|   IBIS model for TI xxx DSP
[IBIS Ver]   5.1
[Disclaimer]   Please be aware that in the absence of a written agreement
|   Texas Instruments(TI) assumes no liability for:
|   (1) The accuracy of the IBIS models provided to your company,
|   however, the IBIS model is compliant to industry standard
|   IQ Level 2a.  Refer to IBIS Quality Section below for
|   for full details.
|   (2) The proper functioning of these Models in your design
|   or for any resulting applications
|   (3) Infringement of patents, copyrights or intellectual
|   property rights resulting from your use of these
|   models.
|   TI provides IBIS Models as a service to our customers and
|   therefore reserves the right to limit distribution of the
|   Models.  The information is subject to change without notice.
[File Name]  sprm785c.ibs
[File Rev]   0.4
|   - Initial version
|   - Fixed typo in I/O assignment
|   - Removed unsupported SDIO/LVCMOS drive strengths
|   - Updated with supported drive strengths for IIC and eMMC buffers
[Date]   26 Oct 2023
[Source]   Texas Instruments Incorporated
[Copyright]   Property of Texas Instruments Incorporated.
|   Unauthorized reproduction and/or distribution is strictly.
|   prohibited.
|   This product is protected under copyright law and trade
|   secret law as an unpublished work.
|   Created 2012,(C) Copyright 1999-2012,
|   Texas Instruments Incorporated., All Rights Reserved.
|   These commodities are under the U.S. Government
|   distribution license control. As such,they are not to be
|   re-exported without the prior approval of the U.S.
|   Department of Commerce.
[Notes]
   This file does not include AMI models for SerDes based links.
   For SerDes simulations use Texas Instruments IBIS AMI models
   Some IV curves contain Non monotonic data points.
|   Revision History
|   GERNERAL COMMENT: All IBIS Quality Notes below reflect latest release
|   and version of IBIS File
|   File passes ibischk5.1 and ibischk6 with 0 errors and 200 warnings
|   Component AM62A
[Component] AM62A
[Manufacturer] Texas Instruments
[Package]
|   typ   min   max
R_pkg   0.40877   0.11887   0.72369
L_pkg   2.422e-9   9.157e-10   3.836e-9
C_pkg   1.228e-12   5.686e-13   1.785e-12
[Package Model]   am62a_pkg
[Pin]	Signal_name	model_name
E7	ATEST0	NC
V11	CSI0_ATB_0_H	NC
U11	CSI0_ATB_1_H	NC
AB14	CSI0_RXCLKN	NC
AB13	CSI0_RXCLKP	NC
W12	CSI0_RXN0	NC
Y13	CSI0_RXN1	NC
AA13	CSI0_RXN2	NC
AB11	CSI0_RXN3	NC
W13	CSI0_RXP0	NC
Y14	CSI0_RXP1	NC
AA12	CSI0_RXP2	NC
AB10	CSI0_RXP3	NC
V10	CSI0_RXRCALIB	NC
J5	DDR0_A0		DDR_SE
J2	DDR0_A1		DDR_SE
K2	DDR0_A10	DDR_SE
L5	DDR0_A11	DDR_SE
M3	DDR0_A12	DDR_SE
M2	DDR0_A13	DDR_SE
J4	DDR0_A2		DDR_SE
L4	DDR0_A3		DDR_SE
J1	DDR0_A4		DDR_SE
K5	DDR0_A5		DDR_SE
K3	DDR0_A6		DDR_SE
H2	DDR0_A7		DDR_SE
L6	DDR0_A8		DDR_SE
L2	DDR0_A9		DDR_SE
N5	DDR0_ACT_N	DDR_SE
H7	DDR0_ALERT_N	DDR_SE
G7	DDR0_ATB0	DDR_SE
F6	DDR0_ATB1	DDR_SE
K6	DDR0_BA0	DDR_SE
H3	DDR0_BA1	DDR_SE
P4	DDR0_BG0	DDR_SE
R7	DDR0_BG1	DDR_SE
H6	DDR0_CAL0	DDR_SE
M5	DDR0_CAS_N	DDR_SE
M1	DDR0_CK0	DDR_DIFF_P
L1	DDR0_CK0_N	DDR_DIFF_N
P3	DDR0_CKE0	DDR_SE
P5	DDR0_CKE1	DDR_SE
J6	DDR0_CS0_N	DDR_SE
N4	DDR0_CS1_N	DDR_SE
C2	DDR0_DM0	DDR_SE
F3	DDR0_DM1	DDR_SE
U1	DDR0_DM2	DDR_SE
W3	DDR0_DM3	DDR_SE
A5	DDR0_DQ0	DDR_SE
B4	DDR0_DQ1	DDR_SE
E6	DDR0_DQ10	DDR_SE
G2	DDR0_DQ11	DDR_SE
G6	DDR0_DQ12	DDR_SE
G4	DDR0_DQ13	DDR_SE
E4	DDR0_DQ14	DDR_SE
D3	DDR0_DQ15	DDR_SE
T6	DDR0_DQ16	DDR_SE
T4	DDR0_DQ17	DDR_SE
U5	DDR0_DQ18	DDR_SE
R5	DDR0_DQ19	DDR_SE
B6	DDR0_DQ2	DDR_SE
P2	DDR0_DQ20	DDR_SE
R3	DDR0_DQ21	DDR_SE
T2	DDR0_DQ22	DDR_SE
U3	DDR0_DQ23	DDR_SE
Y2	DDR0_DQ24	DDR_SE
V2	DDR0_DQ25	DDR_SE
V4	DDR0_DQ26	DDR_SE
W5	DDR0_DQ27	DDR_SE
Y4	DDR0_DQ28	DDR_SE
AA3	DDR0_DQ29	DDR_SE
D5	DDR0_DQ3	DDR_SE
AA5	DDR0_DQ30	DDR_SE
AB4	DDR0_DQ31	DDR_SE
C5	DDR0_DQ4	DDR_SE
C3	DDR0_DQ5	DDR_SE
B2	DDR0_DQ6	DDR_SE
A3	DDR0_DQ7	DDR_SE
E2	DDR0_DQ8	DDR_SE
F5	DDR0_DQ9	DDR_SE
D1	DDR0_DQS0	DDR_DIFF_P
C1	DDR0_DQS0_N	DDR_DIFF_N
G1	DDR0_DQS1	DDR_DIFF_P
F1	DDR0_DQS1_N	DDR_DIFF_N
R1	DDR0_DQS2	DDR_DIFF_P
P1	DDR0_DQS2_N	DDR_DIFF_N
W1	DDR0_DQS3	DDR_DIFF_P
Y1	DDR0_DQS3_N	DDR_DIFF_N
H5	DDR0_ODT0	DDR_SE
N3	DDR0_ODT1	DDR_SE
N2	DDR0_PAR	DDR_SE
M6	DDR0_RAS_N	DDR_SE
P6	DDR0_RESET0_N	DDR_SE
N6	DDR0_WE_N	DDR_SE
C13	EMU0		LVCMOS_V
E10	EMU1		LVCMOS_V
B16	EXT_REFCLK1	LVCMOS_V
F17	EXTINTN		IIC_V
N21	GPMC0_AD0	LVCMOS_H
N20	GPMC0_AD1	LVCMOS_H
R20	GPMC0_AD10	LVCMOS_H
R22	GPMC0_AD11	LVCMOS_H
T22	GPMC0_AD12	LVCMOS_H
R21	GPMC0_AD13	LVCMOS_H
T20	GPMC0_AD14	LVCMOS_H
T21	GPMC0_AD15	LVCMOS_H
N19	GPMC0_AD2	LVCMOS_H
N18	GPMC0_AD3	LVCMOS_H
N17	GPMC0_AD4	LVCMOS_H
P18	GPMC0_AD5	LVCMOS_H
P19	GPMC0_AD6	LVCMOS_H
P21	GPMC0_AD7	LVCMOS_H
P22	GPMC0_AD8	LVCMOS_H
R19	GPMC0_AD9	LVCMOS_H
L18	GPMC0_ADVN_ALE	LVCMOS_H
L19	GPMC0_BE0N_CLE	LVCMOS_H
M18	GPMC0_BE1N	LVCMOS_H
N22	GPMC0_CLK	LVCMOS_H
M19	GPMC0_CSN0	LVCMOS_H
M21	GPMC0_CSN1	LVCMOS_H
M22	GPMC0_CSN2	LVCMOS_H
M20	GPMC0_CSN3	LVCMOS_H
K18	GPMC0_DIR	LVCMOS_H
L17	GPMC0_OEN_REN	LVCMOS_H
R18	GPMC0_WAIT0	LVCMOS_H
R17	GPMC0_WAIT1	LVCMOS_H
K19	GPMC0_WEN	LVCMOS_H
K17	GPMC0_WPN	LVCMOS_H
D17	I2C0_SCL	LVCMOS_V
E16	I2C0_SDA	LVCMOS_V
C17	I2C1_SCL	LVCMOS_V
E17	I2C1_SDA	LVCMOS_V
C6	IFORCE		NC
C18	MCAN0_RX	LVCMOS_V
B17	MCAN0_TX	LVCMOS_V
A21	MCASP0_ACLKR	LVCMOS_V
A19	MCASP0_ACLKX	LVCMOS_V
B21	MCASP0_AFSR	LVCMOS_V
A20	MCASP0_AFSX	LVCMOS_V
B20	MCASP0_AXR0	LVCMOS_V
B18	MCASP0_AXR1	LVCMOS_V
B19	MCASP0_AXR2	LVCMOS_V
C19	MCASP0_AXR3	LVCMOS_V
B8	MCU_ERRORN	LVCMOS_H
E12	MCU_I2C0_SCL	IIC_V
D9	MCU_I2C0_SDA	IIC_V
E8	MCU_MCAN0_RX	LVCMOS_V
C7	MCU_MCAN0_TX	LVCMOS_V
B9	MCU_MCAN1_RX	LVCMOS_V
D7	MCU_MCAN1_TX	LVCMOS_V
A12	MCU_OSC0_XI	NC
A11	MCU_OSC0_XO	NC
A7	MCU_PORZ	RESET_H
D14	MCU_RESETSTATZ	LVCMOS_V
C12	MCU_RESETZ	LVCMOS_V
B13	MCU_SPI0_CLK	LVCMOS_V
E11	MCU_SPI0_CS0	LVCMOS_V
C11	MCU_SPI0_CS1	LVCMOS_V
A15	MCU_SPI0_D0	LVCMOS_V
B12	MCU_SPI0_D1	LVCMOS_V
B11	MCU_UART0_CTSN	LVCMOS_V
D10	MCU_UART0_RTSN	LVCMOS_V
D8	MCU_UART0_RXD	LVCMOS_V
F8	MCU_UART0_TXD	LVCMOS_V
V12	MDIO0_MDC	LVCMOS_V
V13	MDIO0_MDIO	LVCMOS_V
AB7	MMC0_CLK	SDIO_V
Y6	MMC0_CMD	SDIO_V
AA6	MMC0_DAT0	SDIO_V
AB6	MMC0_DAT1	SDIO_V
Y7	MMC0_DAT2	SDIO_V
AA7	MMC0_DAT3	SDIO_V
Y8	MMC0_DAT4	SDIO_V
W7	MMC0_DAT5	SDIO_V
W9	MMC0_DAT6	SDIO_V
AB8	MMC0_DAT7	SDIO_V
E22	MMC1_CLK	SDIO_V
C21	MMC1_CMD	SDIO_V
B22	MMC1_DAT0	SDIO_V
D21	MMC1_DAT1	SDIO_V
C22	MMC1_DAT2	SDIO_V
D22	MMC1_DAT3	SDIO_V
E18	MMC1_SDCD	LVCMOS_V
D18	MMC1_SDWP	LVCMOS_V
H22	MMC2_CLK	SDIO_H
G22	MMC2_CMD	SDIO_H
E20	MMC2_DAT0	SDIO_H
F21	MMC2_DAT1	SDIO_H
F20	MMC2_DAT2	SDIO_H
G21	MMC2_DAT3	SDIO_H
F22	MMC2_SDCD	LVCMOS_H
E21	MMC2_SDWP	LVCMOS_H
L22	OSPI0_CLK	LVCMOS_H
H21	OSPI0_CSN0	LVCMOS_H
G19	OSPI0_CSN1	LVCMOS_H
K20	OSPI0_CSN2	LVCMOS_H
G20	OSPI0_CSN3	LVCMOS_H
J21	OSPI0_D0	LVCMOS_H
J18	OSPI0_D1	LVCMOS_H
J19	OSPI0_D2	LVCMOS_H
H18	OSPI0_D3	LVCMOS_H
K21	OSPI0_D4	LVCMOS_H
H19	OSPI0_D5	LVCMOS_H
J20	OSPI0_D6	LVCMOS_H
J22	OSPI0_D7	LVCMOS_H
L21	OSPI0_DQS	LVCMOS_H
K22	OSPI0_LBCLKO	LVCMOS_H
D12	PMIC_LPM_EN0	LVCMOS_V
F18	PORZ_OUT	LVCMOS_V
E19	RESET_REQZ	LVCMOS_V
F19	RESETSTATZ	LVCMOS_V
AB16	RGMII1_RD0	LVCMOS_V
V15	RGMII1_RD1	LVCMOS_V
W15	RGMII1_RD2	LVCMOS_V
V14	RGMII1_RD3	LVCMOS_V
AA15	RGMII1_RX_CTL	LVCMOS_V
AA16	RGMII1_RXC	LVCMOS_V
Y17	RGMII1_TD0	LVCMOS_V
V16	RGMII1_TD1	LVCMOS_V
Y16	RGMII1_TD2	LVCMOS_V
AA17	RGMII1_TD3	LVCMOS_V
W16	RGMII1_TX_CTL	LVCMOS_V
AB17	RGMII1_TXC	LVCMOS_V
AA21	RGMII2_RD0	LVCMOS_V
Y20	RGMII2_RD1	LVCMOS_V
AB21	RGMII2_RD2	LVCMOS_V
AB20	RGMII2_RD3	LVCMOS_V
W18	RGMII2_RX_CTL	LVCMOS_V
AA20	RGMII2_RXC	LVCMOS_V
AA19	RGMII2_TD0	LVCMOS_V
Y18	RGMII2_TD1	LVCMOS_V
AA18	RGMII2_TD2	LVCMOS_V
W17	RGMII2_TD3	LVCMOS_V
Y19	RGMII2_TX_CTL	LVCMOS_V
AB19	RGMII2_TXC	LVCMOS_V
A17	SPI0_CLK	LVCMOS_V
D16	SPI0_CS0	LVCMOS_V
C16	SPI0_CS1	LVCMOS_V
B15	SPI0_D0		LVCMOS_V
E15	SPI0_D1		LVCMOS_V
A14	TCK		LVCMOS_V
A16	TDI		LVCMOS_V
C14	TDO		LVCMOS_V
F10	TEMP_DIODE_P	NC
B14	TMS		LVCMOS_V
F15	TRSTN		LVCMOS_V
F14	UART0_CTSN	LVCMOS_V
C15	UART0_RTSN	LVCMOS_V
E14	UART0_RXD	LVCMOS_V
D15	UART0_TXD	LVCMOS_V
AA10	USB0_DM		NC
AA9	USB0_DP		NC
C20	USB0_DRVVBUS	LVCMOS_V
W10	USB0_RCALIB	NC
V8	USB0_VBUS	NC
Y11	USB1_DM		NC
Y10	USB1_DP		NC
D19	USB1_DRVVBUS	LVCMOS_V
U7	USB1_RCALIB	NC
V6	USB1_VBUS	NC
U22	VOUT0_DATA0	LVCMOS_H
U21	VOUT0_DATA1	LVCMOS_H
W22	VOUT0_DATA10	LVCMOS_H
W21	VOUT0_DATA11	LVCMOS_H
W20	VOUT0_DATA12	LVCMOS_H
W19	VOUT0_DATA13	LVCMOS_H
Y21	VOUT0_DATA14	LVCMOS_H
Y22	VOUT0_DATA15	LVCMOS_H
U20	VOUT0_DATA2	LVCMOS_H
U19	VOUT0_DATA3	LVCMOS_H
T19	VOUT0_DATA4	LVCMOS_H
U18	VOUT0_DATA5	LVCMOS_H
V22	VOUT0_DATA6	LVCMOS_H
V21	VOUT0_DATA7	LVCMOS_H
V19	VOUT0_DATA8	LVCMOS_H
V18	VOUT0_DATA9	LVCMOS_H
U17	VOUT0_DE	LVCMOS_H
T18	VOUT0_HSYNC	LVCMOS_H
AA22	VOUT0_PCLK	LVCMOS_H
V17	VOUT0_VSYNC	LVCMOS_H
D6	VSENSE		NC
B10	WKUP_CLKOUT0	LVCMOS_V
D13	WKUP_I2C0_SCL	IIC_V
E13	WKUP_I2C0_SDA	IIC_V
A8	WKUP_LFOSC0_XI	NC
A9	WKUP_LFOSC0_XO	NC
C10	WKUP_UART0_CTSN	LVCMOS_V
C8	WKUP_UART0_RTSN	LVCMOS_V
C9	WKUP_UART0_RXD	LVCMOS_V
E9	WKUP_UART0_TXD	LVCMOS_V
A1	VSS	GND
A4	VSS	GND
A6	VSS	GND
A10	VSS	GND
A13	VSS	GND
A18	VSS	GND
A22	VSS	GND
B3	VSS	GND
B5	VSS	GND
B7	VSS	GND
C4	VSS	GND
D2	VSS	GND
D4	VSS	GND
D11	VSS	GND
D20	VSS	GND
E1	VSS	GND
E3	VSS	GND
E5	VSS	GND
F2	VSS	GND
F4	VSS	GND
F11	VSS	GND
F13	VSS	GND
F16	VSS	GND
G3	VSS	GND
G5	VSS	GND
G9	VSS	GND
G12	VSS	GND
G17	VSS	GND
H1	VSS	GND
H4	VSS	GND
H11	VSS	GND
H14	VSS	GND
H20	VSS	GND
J3	VSS	GND
J12	VSS	GND
J17	VSS	GND
K1	VSS	GND
K4	VSS	GND
K7	VSS	GND
K9	VSS	GND
K11	VSS	GND
L3	VSS	GND
L12	VSS	GND
L14	VSS	GND
L20	VSS	GND
M4	VSS	GND
M7	VSS	GND
M11	VSS	GND
M17	VSS	GND
N1	VSS	GND
N8	VSS	GND
N10	VSS	GND
N12	VSS	GND
N14	VSS	GND
N16	VSS	GND
P7	VSS	GND
P11	VSS	GND
P13	VSS	GND
P15	VSS	GND
P17	VSS	GND
P20	VSS	GND
R2	VSS	GND
R4	VSS	GND
R6	VSS	GND
R10	VSS	GND
R12	VSS	GND
R14	VSS	GND
R16	VSS	GND
T1	VSS	GND
T3	VSS	GND
T5	VSS	GND
T7	VSS	GND
T15	VSS	GND
T17	VSS	GND
U2	VSS	GND
U4	VSS	GND
U6	VSS	GND
U9	VSS	GND
U12	VSS	GND
U14	VSS	GND
U16	VSS	GND
V1	VSS	GND
V3	VSS	GND
V5	VSS	GND
V7	VSS	GND
V9	VSS	GND
V20	VSS	GND
W2	VSS	GND
W4	VSS	GND
W6	VSS	GND
W8	VSS	GND
W11	VSS	GND
W14	VSS	GND
Y3	VSS	GND
Y5	VSS	GND
Y9	VSS	GND
Y12	VSS	GND
Y15	VSS	GND
AA2	VSS	GND
AA4	VSS	GND
AA8	VSS	GND
AA11	VSS	GND
AA14	VSS	GND
AB1	VSS	GND
AB3	VSS	GND
AB5	VSS	GND
AB9	VSS	GND
AB12	VSS	GND
AB15	VSS	GND
AB18	VSS	GND
AB22	VSS	GND
G8	CAP_VDDS_CANUART	POWER
G10	CAP_VDDS_MCU	POWER
G13	CAP_VDDS0	POWER
K16	CAP_VDDS1	POWER
T14	CAP_VDDS2	POWER
M16	CAP_VDDS3	POWER
R8	CAP_VDDS4	POWER
G15	CAP_VDDS5	POWER
J16	CAP_VDDS6	POWER
H9	VDD_CANUART	POWER
J9	VDD_CORE	POWER
J11	VDD_CORE	POWER
J13	VDD_CORE	POWER
J15	VDD_CORE	POWER
K14	VDD_CORE	POWER
L9	VDD_CORE	POWER
L11	VDD_CORE	POWER
L13	VDD_CORE	POWER
M12	VDD_CORE	POWER
N11	VDD_CORE	POWER
N13	VDD_CORE	POWER
P10	VDD_CORE	POWER
P14	VDD_CORE	POWER
R9	VDD_CORE	POWER
R15	VDD_CORE	POWER
T16	VDD_CORE	POWER
U15	VDD_CORE	POWER
T12	VDDA_1P8_CSIRX0	POWER
T10	VDDA_1P8_USB	POWER
U10	VDDA_3P3_USB	POWER
T11	VDDA_CORE_CSIRX0	POWER
T9	VDDA_CORE_USB	POWER
M9	VDDA_DDR_PLL0	POWER
J10	VDDA_MCU	POWER
N9	VDDA_PLL0	POWER
R11	VDDA_PLL1	POWER
M13	VDDA_PLL2	POWER
K13	VDDA_PLL3	POWER
K10	VDDA_PLL4	POWER
P16	VDDA_TEMP0	POWER
G18	VDDA_TEMP1	POWER
L10	VDDA_TEMP2	POWER
J14	VDDR_CORE	POWER
K12	VDDR_CORE	POWER
M10	VDDR_CORE	POWER
M14	VDDR_CORE	POWER
P9	VDDR_CORE	POWER
P12	VDDR_CORE	POWER
A2	VDDS_DDR	POWER
B1	VDDS_DDR	POWER
J7	VDDS_DDR	POWER
K8	VDDS_DDR	POWER
L7	VDDS_DDR	POWER
M8	VDDS_DDR	POWER
N7	VDDS_DDR	POWER
P8	VDDS_DDR	POWER
AA1	VDDS_DDR	POWER
AB2	VDDS_DDR	POWER
L8	VDDS_DDR_C	POWER
J8	VDDS_OSC0	POWER
H8	VDDSHV_CANUART	POWER
G11	VDDSHV_MCU	POWER
H10	VDDSHV_MCU	POWER
G14	VDDSHV0	POWER
H13	VDDSHV0	POWER
K15	VDDSHV1	POWER
L16	VDDSHV1	POWER
R13	VDDSHV2	POWER
T13	VDDSHV2	POWER
U13	VDDSHV2	POWER
L15	VDDSHV3	POWER
M15	VDDSHV3	POWER
N15	VDDSHV3	POWER
T8	VDDSHV4	POWER
U8	VDDSHV4	POWER
G16	VDDSHV5	POWER
H15	VDDSHV5	POWER
H16	VDDSHV6	POWER
H17	VDDSHV6	POWER
F12	VMON_1P8_SOC	POWER
F9	VMON_3P3_SOC	POWER
H12	VMON_ER_VSYS	POWER
F7	VPP	POWER
|********************  DIFF PIN  *******************************
[Diff_pin]   inv_pin vdiff tdelay_typ   tdelay_min  tdelay_max
M1	L1	NA	NA	NA	NA	||	DDR0_CK0	&	DDR0_CK0_N
D1	C1	NA	NA	NA	NA	||	DDR0_DQS0	&	DDR0_DQS0_N
G1	F1	NA	NA	NA	NA	||	DDR0_DQS1	&	DDR0_DQS1_N
R1	P1	NA	NA	NA	NA	||	DDR0_DQS2	&	DDR0_DQS2_N
W1	Y1	NA	NA	NA	NA	||	DDR0_DQS3	&	DDR0_DQS3_N
|---------------- DDR -------------------
[Model Selector] DDR_SE
lpddr4_ocd_40p_40n_lt  driver with 40 ohms pullup and 40 ohms pulldown strength, max slew rate
lpddr4_ocd_48p_48n_lt  driver with 48 ohms pullup and 48 ohms pulldown strength, max slew rate
lpddr4_ocd_60p_60n_lt  driver with 60 ohms pullup and 60 ohms pulldown strength, max slew rate
lpddr4_ocd_60p_60n_120pd_lt  driver with 60 ohms pd and 60 ohms pu and 120 pd always on, max slew rate
lpddr4_ocd_80p_80n_lt  driver with 80 ohms pullup and 80 ohms pulldown strength, max slew rate
lpddr4_odt_40_lt  40 ohm termination
lpddr4_odt_48_lt  48 ohm termination
lpddr4_odt_60_lt  60 ohm termination
lpddr4_odt_80_lt  80 ohm termination
lpddr4_odt_120_lt  120 ohm termination
lpddr4_odt_240_lt  240 ohm termination
lpddr4_odt_off_lt  No termination
ddr4_ocd_34p_34n_lt  driver with 34 ohms pullup and 34 ohms pulldown strength, max slew rate
ddr4_ocd_40p_40n_lt  driver with 40 ohms pullup and 40 ohms pulldown strength, max slew rate
ddr4_ocd_48p_48n_lt  driver with 48 ohms pullup and 48 ohms pulldown strength, max slew rate
ddr4_ocd_60p_60n_lt  driver with 60 ohms pullup and 60 ohms pulldown strength, max slew rate
ddr4_ocd_80p_80n_lt  driver with 80 ohms pullup and 80 ohms pulldown strength, max slew rate
ddr4_odt_34_lt  34 ohm termination
ddr4_odt_40_lt  40 ohm termination
ddr4_odt_48_lt  48 ohm termination
ddr4_odt_60_lt  60 ohm termination
ddr4_odt_80_lt  80 ohm termination
ddr4_odt_120_lt  120 ohm termination
ddr4_odt_240_lt  240 ohm termination
ddr4_odt_off_lt  No termination
lpddr4_ocd_40p_40n_ht  driver with 40 ohms pullup and 40 ohms pulldown strength, max slew rate
lpddr4_ocd_48p_48n_ht  driver with 48 ohms pullup and 48 ohms pulldown strength, max slew rate
lpddr4_ocd_60p_60n_ht  driver with 60 ohms pullup and 60 ohms pulldown strength, max slew rate
lpddr4_ocd_60p_60n_120pd_ht  driver with 60 ohms pd and 60 ohms pu and 120 pd always on, max slew rate
lpddr4_ocd_80p_80n_ht  driver with 80 ohms pullup and 80 ohms pulldown strength, max slew rate
lpddr4_odt_40_ht  40 ohm termination
lpddr4_odt_48_ht  48 ohm termination
lpddr4_odt_60_ht  60 ohm termination
lpddr4_odt_80_ht  80 ohm termination
lpddr4_odt_120_ht  120 ohm termination
lpddr4_odt_240_ht  240 ohm termination
lpddr4_odt_off_ht  No termination
ddr4_ocd_34p_34n_ht  driver with 34 ohms pullup and 34 ohms pulldown strength, max slew rate
ddr4_ocd_40p_40n_ht  driver with 40 ohms pullup and 40 ohms pulldown strength, max slew rate
ddr4_ocd_48p_48n_ht  driver with 48 ohms pullup and 48 ohms pulldown strength, max slew rate
ddr4_ocd_60p_60n_ht  driver with 60 ohms pullup and 60 ohms pulldown strength, max slew rate
ddr4_ocd_80p_80n_ht  driver with 80 ohms pullup and 80 ohms pulldown strength, max slew rate
ddr4_odt_34_ht  34 ohm termination
ddr4_odt_40_ht  40 ohm termination
ddr4_odt_48_ht  48 ohm termination
ddr4_odt_60_ht  60 ohm termination
ddr4_odt_80_ht  80 ohm termination
ddr4_odt_120_ht  120 ohm termination
ddr4_odt_240_ht  240 ohm termination
ddr4_odt_off_ht  No termination
[Model Selector] DDR_DIFF_P
lpddr4_ocd_40p_40n_p_lt  driver with 40 ohms pullup and 40 ohms pulldown strength, max slew rate
lpddr4_ocd_48p_48n_p_lt  driver with 48 ohms pullup and 48 ohms pulldown strength, max slew rate
lpddr4_ocd_60p_60n_p_lt  driver with 60 ohms pullup and 60 ohms pulldown strength, max slew rate
lpddr4_ocd_60p_60n_120pd_p_lt  driver with 60 ohms pd and 60 ohms pu and 120 pd always on, max slew rate
lpddr4_ocd_80p_80n_p_lt  driver with 80 ohms pullup and 80 ohms pulldown strength, max slew rate
lpddr4_odt_40_diff_lt  40 ohm termination
lpddr4_odt_48_diff_lt  48 ohm termination
lpddr4_odt_60_diff_lt  60 ohm termination
lpddr4_odt_80_diff_lt  80 ohm termination
lpddr4_odt_120_diff_lt  120 ohm termination
lpddr4_odt_240_diff_lt  240 ohm termination
lpddr4_odt_off_diff_lt  No termination
ddr4_ocd_34p_34n_P_lt  driver with 34 ohms pullup and 34 ohms pulldown strength, max slew rate
ddr4_ocd_40p_40n_P_lt  driver with 40 ohms pullup and 40 ohms pulldown strength, max slew rate
ddr4_ocd_48p_48n_P_lt  driver with 48 ohms pullup and 48 ohms pulldown strength, max slew rate
ddr4_ocd_60p_60n_P_lt  driver with 60 ohms pullup and 60 ohms pulldown strength, max slew rate
ddr4_ocd_80p_80n_P_lt  driver with 80 ohms pullup and 80 ohms pulldown strength, max slew rate
ddr4_odt_34_diff_lt  34 ohm termination
ddr4_odt_40_diff_lt  40 ohm termination
ddr4_odt_48_diff_lt  48 ohm termination
ddr4_odt_60_diff_lt  60 ohm termination
ddr4_odt_80_diff_lt  80 ohm termination
ddr4_odt_120_diff_lt  120 ohm termination
ddr4_odt_240_diff_lt  240 ohm termination
ddr4_odt_off_diff_lt  No termination
lpddr4_ocd_40p_40n_p_ht  driver with 40 ohms pullup and 40 ohms pulldown strength, max slew rate
lpddr4_ocd_48p_48n_p_ht  driver with 48 ohms pullup and 48 ohms pulldown strength, max slew rate
lpddr4_ocd_60p_60n_p_ht  driver with 60 ohms pullup and 60 ohms pulldown strength, max slew rate
lpddr4_ocd_60p_60n_120pd_p_ht  driver with 60 ohms pd and 60 ohms pu and 120 pd always on, max slew rate
lpddr4_ocd_80p_80n_p_ht  driver with 80 ohms pullup and 80 ohms pulldown strength, max slew rate
lpddr4_odt_40_diff_ht  40 ohm termination
lpddr4_odt_48_diff_ht  48 ohm termination
lpddr4_odt_60_diff_ht  60 ohm termination
lpddr4_odt_80_diff_ht  80 ohm termination
lpddr4_odt_120_diff_ht  120 ohm termination
lpddr4_odt_240_diff_ht  240 ohm termination
lpddr4_odt_off_diff_ht  No termination
ddr4_ocd_34p_34n_P_ht  driver with 34 ohms pullup and 34 ohms pulldown strength, max slew rate
ddr4_ocd_40p_40n_P_ht  driver with 40 ohms pullup and 40 ohms pulldown strength, max slew rate
ddr4_ocd_48p_48n_P_ht  driver with 48 ohms pullup and 48 ohms pulldown strength, max slew rate
ddr4_ocd_60p_60n_P_ht  driver with 60 ohms pullup and 60 ohms pulldown strength, max slew rate
ddr4_ocd_80p_80n_P_ht  driver with 80 ohms pullup and 80 ohms pulldown strength, max slew rate
ddr4_odt_34_diff_ht  34 ohm termination
ddr4_odt_40_diff_ht  40 ohm termination
ddr4_odt_48_diff_ht  48 ohm termination
ddr4_odt_60_diff_ht  60 ohm termination
ddr4_odt_80_diff_ht  80 ohm termination
ddr4_odt_120_diff_ht  120 ohm termination
ddr4_odt_240_diff_ht  240 ohm termination
ddr4_odt_off_diff_ht  No termination
[Model Selector] DDR_DIFF_N
lpddr4_ocd_40p_40n_n_lt  driver with 40 ohms pullup and 40 ohms pulldown strength, max slew rate
lpddr4_ocd_48p_48n_n_lt  driver with 48 ohms pullup and 48 ohms pulldown strength, max slew rate
lpddr4_ocd_60p_60n_n_lt  driver with 60 ohms pullup and 60 ohms pulldown strength, max slew rate
lpddr4_ocd_60p_60n_120pd_n_lt  driver with 60 ohms pd and 60 ohms pu and 120 pd always on, max slew rate
lpddr4_ocd_80p_80n_n_lt  driver with 80 ohms pullup and 80 ohms pulldown strength, max slew rate
lpddr4_odt_40_diff_lt  40 ohm termination
lpddr4_odt_48_diff_lt  48 ohm termination
lpddr4_odt_60_diff_lt  60 ohm termination
lpddr4_odt_80_diff_lt  80 ohm termination
lpddr4_odt_120_diff_lt  120 ohm termination
lpddr4_odt_240_diff_lt  240 ohm termination
lpddr4_odt_off_diff_lt  No termination
ddr4_ocd_34p_34n_N_lt  driver with 34 ohms pullup and 34 ohms pulldown strength, max slew rate
ddr4_ocd_40p_40n_N_lt  driver with 40 ohms pullup and 40 ohms pulldown strength, max slew rate
ddr4_ocd_48p_48n_N_lt  driver with 48 ohms pullup and 48 ohms pulldown strength, max slew rate
ddr4_ocd_60p_60n_N_lt  driver with 60 ohms pullup and 60 ohms pulldown strength, max slew rate
ddr4_ocd_80p_80n_N_lt  driver with 80 ohms pullup and 80 ohms pulldown strength, max slew rate
ddr4_odt_34_diff_lt  34 ohm termination
ddr4_odt_40_diff_lt  40 ohm termination
ddr4_odt_48_diff_lt  48 ohm termination
ddr4_odt_60_diff_lt  60 ohm termination
ddr4_odt_80_diff_lt  80 ohm termination
ddr4_odt_120_diff_lt  120 ohm termination
ddr4_odt_240_diff_lt  240 ohm termination
ddr4_odt_off_diff_lt  No termination
lpddr4_ocd_40p_40n_n_ht  driver with 40 ohms pullup and 40 ohms pulldown strength, max slew rate
lpddr4_ocd_48p_48n_n_ht  driver with 48 ohms pullup and 48 ohms pulldown strength, max slew rate
lpddr4_ocd_60p_60n_n_ht  driver with 60 ohms pullup and 60 ohms pulldown strength, max slew rate
lpddr4_ocd_60p_60n_120pd_n_ht  driver with 60 ohms pd and 60 ohms pu and 120 pd always on, max slew rate
lpddr4_ocd_80p_80n_n_ht  driver with 80 ohms pullup and 80 ohms pulldown strength, max slew rate
lpddr4_odt_40_diff_ht  40 ohm termination
lpddr4_odt_48_diff_ht  48 ohm termination
lpddr4_odt_60_diff_ht  60 ohm termination
lpddr4_odt_80_diff_ht  80 ohm termination
lpddr4_odt_120_diff_ht  120 ohm termination
lpddr4_odt_240_diff_ht  240 ohm termination
lpddr4_odt_off_diff_ht  No termination
ddr4_ocd_34p_34n_N_ht  driver with 34 ohms pullup and 34 ohms pulldown strength, max slew rate
ddr4_ocd_40p_40n_N_ht  driver with 40 ohms pullup and 40 ohms pulldown strength, max slew rate
ddr4_ocd_48p_48n_N_ht  driver with 48 ohms pullup and 48 ohms pulldown strength, max slew rate
ddr4_ocd_60p_60n_N_ht  driver with 60 ohms pullup and 60 ohms pulldown strength, max slew rate
ddr4_ocd_80p_80n_N_ht  driver with 80 ohms pullup and 80 ohms pulldown strength, max slew rate
ddr4_odt_34_diff_ht  34 ohm termination
ddr4_odt_40_diff_ht  40 ohm termination
ddr4_odt_48_diff_ht  48 ohm termination
ddr4_odt_60_diff_ht  60 ohm termination
ddr4_odt_80_diff_ht  80 ohm termination
ddr4_odt_120_diff_ht  120 ohm termination
ddr4_odt_240_diff_ht  240 ohm termination
ddr4_odt_off_diff_ht  No termination
|****************** SDIO
[Model Selector] SDIO_H
sdio1_r40_1p8_h PRWDWUWSWEWCDGSDIO_H@_R40_1p8_comment
sdio1_r40_3p3_h PRWDWUWSWEWCDGSDIO_H@_R40_3p3_comment
[Model Selector] SDIO_V
sdio0_r40_1p8_v PRWDWUWSWEWCDGSDIO_V@_R40_1p8_comment
sdio0_r40_3p3_v PRWDWUWSWEWCDGSDIO_V@_R40_3p3_comment
|********** LVCMOS
[Model Selector] LVCMOS_H
lvcmos1_nom_1p8_h PRWDWUWSWEWCDGLVCMOS_H@_Nom_1p8_comment
lvcmos1_nom_3p3_h PRWDWUWSWEWCDGLVCMOS_H@_Nom_3p3_comment
[Model Selector] LVCMOS_V
lvcmos0_nom_1p8_v PRWDWUWSWEWCDGLVCMOS_V@_Nom_1p8_comment
lvcmos0_nom_3p3_v PRWDWUWSWEWCDGLVCMOS_V@_Nom_3p3_comment
[Model Selector] IIC_V
IIC18_1_0_V PRBOPDDGZIIC_V@HSMODE_HSMCSE=0_0_comment 1.8V
IIC18_1_1_V PRBOPDDGZIIC_V@HSMODE_HSMCSE=0_1_comment 1.8V
IIC18_1_2_V PRBOPDDGZIIC_V@HSMODE_HSMCSE=1_0_comment 1.8V
IIC18_1_3_V PRBOPDDGZIIC_V@HSMODE_HSMCSE=1_1_comment 1.8V
IIC33_1_0_V PRBOPDDGZIIC_V@HSMODE_HSMCSE=0_0_comment
[Model Selector] LVDS
lvds_tx_03   LVDS TX Driver Permumentation 03
lvds_tx_11   LVDS TX Driver Permumentation 11
|***************** RESET ************************************************
[Model Selector] RESET_H
reset18_0_0 PDIDGZRESET_H
|   EMMC
[MODEL SELECTOR] EMMC
emmc51_io_tx40ohm   40ohm DRIVER
|   Package Model
[Define Package Model]   am62a_pkg
[Manufacturer]   name 1
[OEM]   name 2
[Description]   333-pin Package
|[Number of Sections]   1
[Number of Pins]   333
[Pin Numbers]
|[Pin Name]  Net Number   Net Name   Net's All Pins
G13   | 1   CAP_VDDS0   G13
K16   | 2   CAP_VDDS1   K16
T14   | 3   CAP_VDDS2   T14
M16   | 4   CAP_VDDS3   M16
R8   | 5   CAP_VDDS4   R8
G15   | 6   CAP_VDDS5   G15
J16   | 7   CAP_VDDS6   J16
G8   | 8   CAP_VDDS_CANUART   G8
G10   | 9   CAP_VDDS_MCU   G10
T12   | 10   VDDA_1P8_CSIRX0   T12
T10   | 11   VDDA_1P8_USB   T10
U10   | 12   VDDA_3P3_USB   U10
T11   | 13   VDDA_CORE_CSIRX0   T11
T9   | 14   VDDA_CORE_USB   T9
M9   | 15   VDDA_DDR_PLL0   M9
J10   | 16   VDDA_MCU   J10
N9   | 17   VDDA_PLL0   N9
R11   | 18   VDDA_PLL1   R11
M13   | 19   VDDA_PLL2   M13
K13   | 20   VDDA_PLL3   K13
K10   | 21   VDDA_PLL4   K10
P16   | 22   VDDA_TEMP0   P16
G18   | 23   VDDA_TEMP1   G18
L10   | 24   VDDA_TEMP2   L10
P9   | 25   VDDR_CORE   P9
   |P12
   |M14
   |M10
   |K12
   |J14
H13   | 26   VDDSHV0   H13
   |G14
L16   | 27   VDDSHV1   L16
   |K15
U13   | 28   VDDSHV2   U13
   |T13
   |R13
N15   | 29   VDDSHV3   N15
   |M15
   |L15
U8   | 30   VDDSHV4   U8
   |T8
H15   | 31   VDDSHV5   H15
   |G16
H17   | 32   VDDSHV6   H17
   |H16
H8   | 33   VDDSHV_CANUART   H8
H10   | 34   VDDSHV_MCU   H10
   |G11
P8   | 35   VDDS_DDR   P8
   |N7
   |M8
   |L7
   |K8
   |J7
   |B1
   |AB2
   |AA1
   |A2
L8   | 36   VDDS_DDR_C   L8
J8   | 37   VDDS_OSC0   J8
H9   | 38   VDD_CANUART   H9
U15   | 39   VDD_CORE   U15
   |T16
   |R9
   |R15
   |P14
   |P10
   |N13
   |N11
   |M12
   |L9
   |L13
   |L11
   |K14
   |J9
   |J15
   |J13
   |J11
F7   | 40   VPP   F7
E7   | 41   ATEST0   E7
V11   | 42   CSI0_ATB_0_H   V11
U11   | 43   CSI0_ATB_1_H   U11
AB14   | 44   CSI0_RXCLKN   AB14
AB13   | 45   CSI0_RXCLKP   AB13
W12   | 46   CSI0_RXN0   W12
Y13   | 47   CSI0_RXN1   Y13
AA13   | 48   CSI0_RXN2   AA13
AB11   | 49   CSI0_RXN3   AB11
W13   | 50   CSI0_RXP0   W13
Y14   | 51   CSI0_RXP1   Y14
AA12   | 52   CSI0_RXP2   AA12
AB10   | 53   CSI0_RXP3   AB10
V10   | 54   CSI0_RXRCALIB   V10
J5   | 55   DDR0_A0   J5
J2   | 56   DDR0_A1   J2
J4   | 57   DDR0_A2   J4
L4   | 58   DDR0_A3   L4
J1   | 59   DDR0_A4   J1
K5   | 60   DDR0_A5   K5
K3   | 61   DDR0_A6   K3
H2   | 62   DDR0_A7   H2
L6   | 63   DDR0_A8   L6
L2   | 64   DDR0_A9   L2
K2   | 65   DDR0_A10   K2
L5   | 66   DDR0_A11   L5
M3   | 67   DDR0_A12   M3
M2   | 68   DDR0_A13   M2
N5   | 69   DDR0_ACT_N   N5
H7   | 70   DDR0_ALERT_N   H7
G7   | 71   DDR0_ATB0   G7
F6   | 72   DDR0_ATB1   F6
K6   | 73   DDR0_BA0   K6
H3   | 74   DDR0_BA1   H3
P4   | 75   DDR0_BG0   P4
R7   | 76   DDR0_BG1   R7
H6   | 77   DDR0_CAL0   H6
M5   | 78   DDR0_CAS_N   M5
M1   | 79   DDR0_CK0   M1
L1   | 80   DDR0_CK0_N   L1
P3   | 81   DDR0_CKE0   P3
P5   | 82   DDR0_CKE1   P5
J6   | 83   DDR0_CS0_N   J6
N4   | 84   DDR0_CS1_N   N4
C2   | 85   DDR0_DM0   C2
F3   | 86   DDR0_DM1   F3
U1   | 87   DDR0_DM2   U1
W3   | 88   DDR0_DM3   W3
A5   | 89   DDR0_DQ0   A5
B4   | 90   DDR0_DQ1   B4
B6   | 91   DDR0_DQ2   B6
D5   | 92   DDR0_DQ3   D5
C5   | 93   DDR0_DQ4   C5
C3   | 94   DDR0_DQ5   C3
B2   | 95   DDR0_DQ6   B2
A3   | 96   DDR0_DQ7   A3
E2   | 97   DDR0_DQ8   E2
F5   | 98   DDR0_DQ9   F5
E6   | 99   DDR0_DQ10   E6
G2   | 100   DDR0_DQ11   G2
G6   | 101   DDR0_DQ12   G6
G4   | 102   DDR0_DQ13   G4
E4   | 103   DDR0_DQ14   E4
D3   | 104   DDR0_DQ15   D3
T6   | 105   DDR0_DQ16   T6
T4   | 106   DDR0_DQ17   T4
U5   | 107   DDR0_DQ18   U5
R5   | 108   DDR0_DQ19   R5
P2   | 109   DDR0_DQ20   P2
R3   | 110   DDR0_DQ21   R3
T2   | 111   DDR0_DQ22   T2
U3   | 112   DDR0_DQ23   U3
Y2   | 113   DDR0_DQ24   Y2
V2   | 114   DDR0_DQ25   V2
V4   | 115   DDR0_DQ26   V4
W5   | 116   DDR0_DQ27   W5
Y4   | 117   DDR0_DQ28   Y4
AA3   | 118   DDR0_DQ29   AA3
AA5   | 119   DDR0_DQ30   AA5
AB4   | 120   DDR0_DQ31   AB4
D1   | 121   DDR0_DQS0   D1
C1   | 122   DDR0_DQS0_N   C1
G1   | 123   DDR0_DQS1   G1
F1   | 124   DDR0_DQS1_N   F1
R1   | 125   DDR0_DQS2   R1
P1   | 126   DDR0_DQS2_N   P1
W1   | 127   DDR0_DQS3   W1
Y1   | 128   DDR0_DQS3_N   Y1
H5   | 129   DDR0_ODT0   H5
N3   | 130   DDR0_ODT1   N3
N2   | 131   DDR0_PAR   N2
M6   | 132   DDR0_RAS_N   M6
P6   | 133   DDR0_RESET0_N   P6
N6   | 134   DDR0_WE_N   N6
C13   | 135   EMU0   C13
E10   | 136   EMU1   E10
F17   | 137   EXTINTN   F17
B16   | 138   EXT_REFCLK1   B16
N21   | 139   GPMC0_AD0   N21
N20   | 140   GPMC0_AD1   N20
N19   | 141   GPMC0_AD2   N19
N18   | 142   GPMC0_AD3   N18
N17   | 143   GPMC0_AD4   N17
P18   | 144   GPMC0_AD5   P18
P19   | 145   GPMC0_AD6   P19
P21   | 146   GPMC0_AD7   P21
P22   | 147   GPMC0_AD8   P22
R19   | 148   GPMC0_AD9   R19
R20   | 149   GPMC0_AD10   R20
R22   | 150   GPMC0_AD11   R22
T22   | 151   GPMC0_AD12   T22
R21   | 152   GPMC0_AD13   R21
T20   | 153   GPMC0_AD14   T20
T21   | 154   GPMC0_AD15   T21
L18   | 155   GPMC0_ADVN_ALE   L18
L19   | 156   GPMC0_BE0N_CLE   L19
M18   | 157   GPMC0_BE1N   M18
N22   | 158   GPMC0_CLK   N22
M19   | 159   GPMC0_CSN0   M19
M21   | 160   GPMC0_CSN1   M21
M22   | 161   GPMC0_CSN2   M22
M20   | 162   GPMC0_CSN3   M20
K18   | 163   GPMC0_DIR   K18
L17   | 164   GPMC0_OEN_REN   L17
R18   | 165   GPMC0_WAIT0   R18
R17   | 166   GPMC0_WAIT1   R17
K19   | 167   GPMC0_WEN   K19
K17   | 168   GPMC0_WPN   K17
D17   | 169   I2C0_SCL   D17
E16   | 170   I2C0_SDA   E16
C17   | 171   I2C1_SCL   C17
E17   | 172   I2C1_SDA   E17
C6   | 173   IFORCE   C6
C18   | 174   MCAN0_RX   C18
B17   | 175   MCAN0_TX   B17
A21   | 176   MCASP0_ACLKR   A21
A19   | 177   MCASP0_ACLKX   A19
B21   | 178   MCASP0_AFSR   B21
A20   | 179   MCASP0_AFSX   A20
B20   | 180   MCASP0_AXR0   B20
B18   | 181   MCASP0_AXR1   B18
B19   | 182   MCASP0_AXR2   B19
C19   | 183   MCASP0_AXR3   C19
B8   | 184   MCU_ERRORN   B8
E12   | 185   MCU_I2C0_SCL   E12
D9   | 186   MCU_I2C0_SDA   D9
E8   | 187   MCU_MCAN0_RX   E8
C7   | 188   MCU_MCAN0_TX   C7
B9   | 189   MCU_MCAN1_RX   B9
D7   | 190   MCU_MCAN1_TX   D7
A12   | 191   MCU_OSC0_XI   A12
A11   | 192   MCU_OSC0_XO   A11
A7   | 193   MCU_PORZ   A7
D14   | 194   MCU_RESETSTATZ   D14
C12   | 195   MCU_RESETZ   C12
B13   | 196   MCU_SPI0_CLK   B13
E11   | 197   MCU_SPI0_CS0   E11
C11   | 198   MCU_SPI0_CS1   C11
A15   | 199   MCU_SPI0_D0   A15
B12   | 200   MCU_SPI0_D1   B12
B11   | 201   MCU_UART0_CTSN   B11
D10   | 202   MCU_UART0_RTSN   D10
D8   | 203   MCU_UART0_RXD   D8
F8   | 204   MCU_UART0_TXD   F8
V12   | 205   MDIO0_MDC   V12
V13   | 206   MDIO0_MDIO   V13
AB7   | 207   MMC0_CLK   AB7
Y6   | 208   MMC0_CMD   Y6
AA6   | 209   MMC0_DAT0   AA6
AB6   | 210   MMC0_DAT1   AB6
Y7   | 211   MMC0_DAT2   Y7
AA7   | 212   MMC0_DAT3   AA7
Y8   | 213   MMC0_DAT4   Y8
W7   | 214   MMC0_DAT5   W7
W9   | 215   MMC0_DAT6   W9
AB8   | 216   MMC0_DAT7   AB8
E22   | 217   MMC1_CLK   E22
C21   | 218   MMC1_CMD   C21
B22   | 219   MMC1_DAT0   B22
D21   | 220   MMC1_DAT1   D21
C22   | 221   MMC1_DAT2   C22
D22   | 222   MMC1_DAT3   D22
E18   | 223   MMC1_SDCD   E18
D18   | 224   MMC1_SDWP   D18
H22   | 225   MMC2_CLK   H22
G22   | 226   MMC2_CMD   G22
E20   | 227   MMC2_DAT0   E20
F21   | 228   MMC2_DAT1   F21
F20   | 229   MMC2_DAT2   F20
G21   | 230   MMC2_DAT3   G21
F22   | 231   MMC2_SDCD   F22
E21   | 232   MMC2_SDWP   E21
L22   | 233   OSPI0_CLK   L22
H21   | 234   OSPI0_CSN0   H21
G19   | 235   OSPI0_CSN1   G19
K20   | 236   OSPI0_CSN2   K20
G20   | 237   OSPI0_CSN3   G20
J21   | 238   OSPI0_D0   J21
J18   | 239   OSPI0_D1   J18
J19   | 240   OSPI0_D2   J19
H18   | 241   OSPI0_D3   H18
K21   | 242   OSPI0_D4   K21
H19   | 243   OSPI0_D5   H19
J20   | 244   OSPI0_D6   J20
J22   | 245   OSPI0_D7   J22
L21   | 246   OSPI0_DQS   L21
K22   | 247   OSPI0_LBCLKO   K22
D12   | 248   PMIC_LPM_EN0   D12
F18   | 249   PORZ_OUT   F18
F19   | 250   RESETSTATZ   F19
E19   | 251   RESET_REQZ   E19
AB16   | 252   RGMII1_RD0   AB16
V15   | 253   RGMII1_RD1   V15
W15   | 254   RGMII1_RD2   W15
V14   | 255   RGMII1_RD3   V14
AA16   | 256   RGMII1_RXC   AA16
AA15   | 257   RGMII1_RX_CTL   AA15
Y17   | 258   RGMII1_TD0   Y17
V16   | 259   RGMII1_TD1   V16
Y16   | 260   RGMII1_TD2   Y16
AA17   | 261   RGMII1_TD3   AA17
AB17   | 262   RGMII1_TXC   AB17
W16   | 263   RGMII1_TX_CTL   W16
AA21   | 264   RGMII2_RD0   AA21
Y20   | 265   RGMII2_RD1   Y20
AB21   | 266   RGMII2_RD2   AB21
AB20   | 267   RGMII2_RD3   AB20
AA20   | 268   RGMII2_RXC   AA20
W18   | 269   RGMII2_RX_CTL   W18
AA19   | 270   RGMII2_TD0   AA19
Y18   | 271   RGMII2_TD1   Y18
AA18   | 272   RGMII2_TD2   AA18
W17   | 273   RGMII2_TD3   W17
AB19   | 274   RGMII2_TXC   AB19
Y19   | 275   RGMII2_TX_CTL   Y19
A17   | 276   SPI0_CLK   A17
D16   | 277   SPI0_CS0   D16
C16   | 278   SPI0_CS1   C16
B15   | 279   SPI0_D0   B15
E15   | 280   SPI0_D1   E15
A14   | 281   TCK   A14
A16   | 282   TDI   A16
C14   | 283   TDO   C14
F10   | 284   TEMP_DIODE_P   F10
B14   | 285   TMS   B14
F15   | 286   TRSTN   F15
F14   | 287   UART0_CTSN   F14
C15   | 288   UART0_RTSN   C15
E14   | 289   UART0_RXD   E14
D15   | 290   UART0_TXD   D15
AA10   | 291   USB0_DM   AA10
AA9   | 292   USB0_DP   AA9
C20   | 293   USB0_DRVVBUS   C20
W10   | 294   USB0_RCALIB   W10
V8   | 295   USB0_VBUS   V8
Y11   | 296   USB1_DM   Y11
Y10   | 297   USB1_DP   Y10
D19   | 298   USB1_DRVVBUS   D19
U7   | 299   USB1_RCALIB   U7
V6   | 300   USB1_VBUS   V6
F12   | 301   VMON_1P8_SOC   F12
F9   | 302   VMON_3P3_SOC   F9
H12   | 303   VMON_ER_VSYS   H12
U22   | 304   VOUT0_DATA0   U22
U21   | 305   VOUT0_DATA1   U21
U20   | 306   VOUT0_DATA2   U20
U19   | 307   VOUT0_DATA3   U19
T19   | 308   VOUT0_DATA4   T19
U18   | 309   VOUT0_DATA5   U18
V22   | 310   VOUT0_DATA6   V22
V21   | 311   VOUT0_DATA7   V21
V19   | 312   VOUT0_DATA8   V19
V18   | 313   VOUT0_DATA9   V18
W22   | 314   VOUT0_DATA10   W22
W21   | 315   VOUT0_DATA11   W21
W20   | 316   VOUT0_DATA12   W20
W19   | 317   VOUT0_DATA13   W19
Y21   | 318   VOUT0_DATA14   Y21
Y22   | 319   VOUT0_DATA15   Y22
U17   | 320   VOUT0_DE   U17
T18   | 321   VOUT0_HSYNC   T18
AA22   | 322   VOUT0_PCLK   AA22
V17   | 323   VOUT0_VSYNC   V17
D6   | 324   VSENSE   D6
B10   | 325   WKUP_CLKOUT0   B10
D13   | 326   WKUP_I2C0_SCL   D13
E13   | 327   WKUP_I2C0_SDA   E13
A8   | 328   WKUP_LFOSC0_XI   A8
A9   | 329   WKUP_LFOSC0_XO   A9
C10   | 330   WKUP_UART0_CTSN   C10
C8   | 331   WKUP_UART0_RTSN   C8
C9   | 332   WKUP_UART0_RXD   C9
E9   | 333   WKUP_UART0_TXD   E9
[Model Data]
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[End Model Data]
[End Package Model]
| Models and submodels in the file (189): lvcmos1_nom_1p8_h (I/O), lvcmos0_nom_1p8_v (I/O), lvcmos1_nom_3p3_h (I/O), lvcmos0_nom_3p3_v (I/O), lvcmos1_slow_1p8_h (I/O), lvcmos0_slow_1p8_v (I/O), lvcmos1_slow_3p3_h (I/O), lvcmos0_slow_3p3_v (I/O), lvcmos1_fast_1p8_h (I/O), lvcmos0_fast_1p8_v (I/O), lvcmos1_fast_3p3_h (I/O), lvcmos0_fast_3p3_v (I/O), sdio1_r33_1p8_h (I/O), sdio0_r33_1p8_v (I/O), sdio1_r33_3p3_h (I/O), sdio0_r33_3p3_v (I/O), sdio1_r40_1p8_h (I/O), sdio0_r40_1p8_v (I/O), sdio1_r40_3p3_h (I/O), sdio0_r40_3p3_v (I/O), sdio1_r50_1p8_h (I/O), sdio0_r50_1p8_v (I/O), sdio1_r50_3p3_h (I/O), sdio0_r50_3p3_v (I/O), sdio1_r66_1p8_h (I/O), sdio0_r66_1p8_v (I/O), sdio1_r66_3p3_h (I/O), sdio0_r66_3p3_v (I/O), lpddr4_ocd_40p_40n_lt (I/O), lpddr4_ocd_48p_48n_lt (I/O), lpddr4_ocd_60p_60n_lt (I/O), lpddr4_ocd_60p_60n_120pd_lt (I/O), lpddr4_ocd_80p_80n_lt (I/O), lpddr4_ocd_40p_40n_p_lt (I/O), lpddr4_ocd_40p_40n_n_lt (I/O), lpddr4_ocd_48p_48n_p_lt (I/O), lpddr4_ocd_48p_48n_n_lt (I/O), lpddr4_ocd_60p_60n_p_lt (I/O), lpddr4_ocd_60p_60n_n_lt (I/O), lpddr4_ocd_60p_60n_120pd_p_lt (I/O), lpddr4_ocd_60p_60n_120pd_n_lt (I/O), lpddr4_ocd_80p_80n_p_lt (I/O), lpddr4_ocd_80p_80n_n_lt (I/O), lpddr4_odt_40_lt (Input), lpddr4_odt_48_lt (Input), lpddr4_odt_60_lt (Input), lpddr4_odt_80_lt (Input), lpddr4_odt_120_lt (Input), lpddr4_odt_240_lt (Input), lpddr4_odt_off_lt (Input), lpddr4_odt_40_diff_lt (Input), lpddr4_odt_48_diff_lt (Input), lpddr4_odt_60_diff_lt (Input), lpddr4_odt_80_diff_lt (Input), lpddr4_odt_120_diff_lt (Input), lpddr4_odt_240_diff_lt (Input), lpddr4_odt_off_diff_lt (Input), lpddr4_ocd_40p_40n_ht (I/O), lpddr4_ocd_48p_48n_ht (I/O), lpddr4_ocd_60p_60n_ht (I/O), lpddr4_ocd_60p_60n_120pd_ht (I/O), lpddr4_ocd_80p_80n_ht (I/O), lpddr4_ocd_40p_40n_p_ht (I/O), lpddr4_ocd_40p_40n_n_ht (I/O), lpddr4_ocd_48p_48n_p_ht (I/O), lpddr4_ocd_48p_48n_n_ht (I/O), lpddr4_ocd_60p_60n_p_ht (I/O), lpddr4_ocd_60p_60n_n_ht (I/O), lpddr4_ocd_60p_60n_120pd_p_ht (I/O), lpddr4_ocd_60p_60n_120pd_n_ht (I/O), lpddr4_ocd_80p_80n_p_ht (I/O), lpddr4_ocd_80p_80n_n_ht (I/O), lpddr4_odt_40_ht (Input), lpddr4_odt_48_ht (Input), lpddr4_odt_60_ht (Input), lpddr4_odt_80_ht (Input), lpddr4_odt_120_ht (Input), lpddr4_odt_240_ht (Input), lpddr4_odt_off_ht (Input), lpddr4_odt_40_diff_ht (Input)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
